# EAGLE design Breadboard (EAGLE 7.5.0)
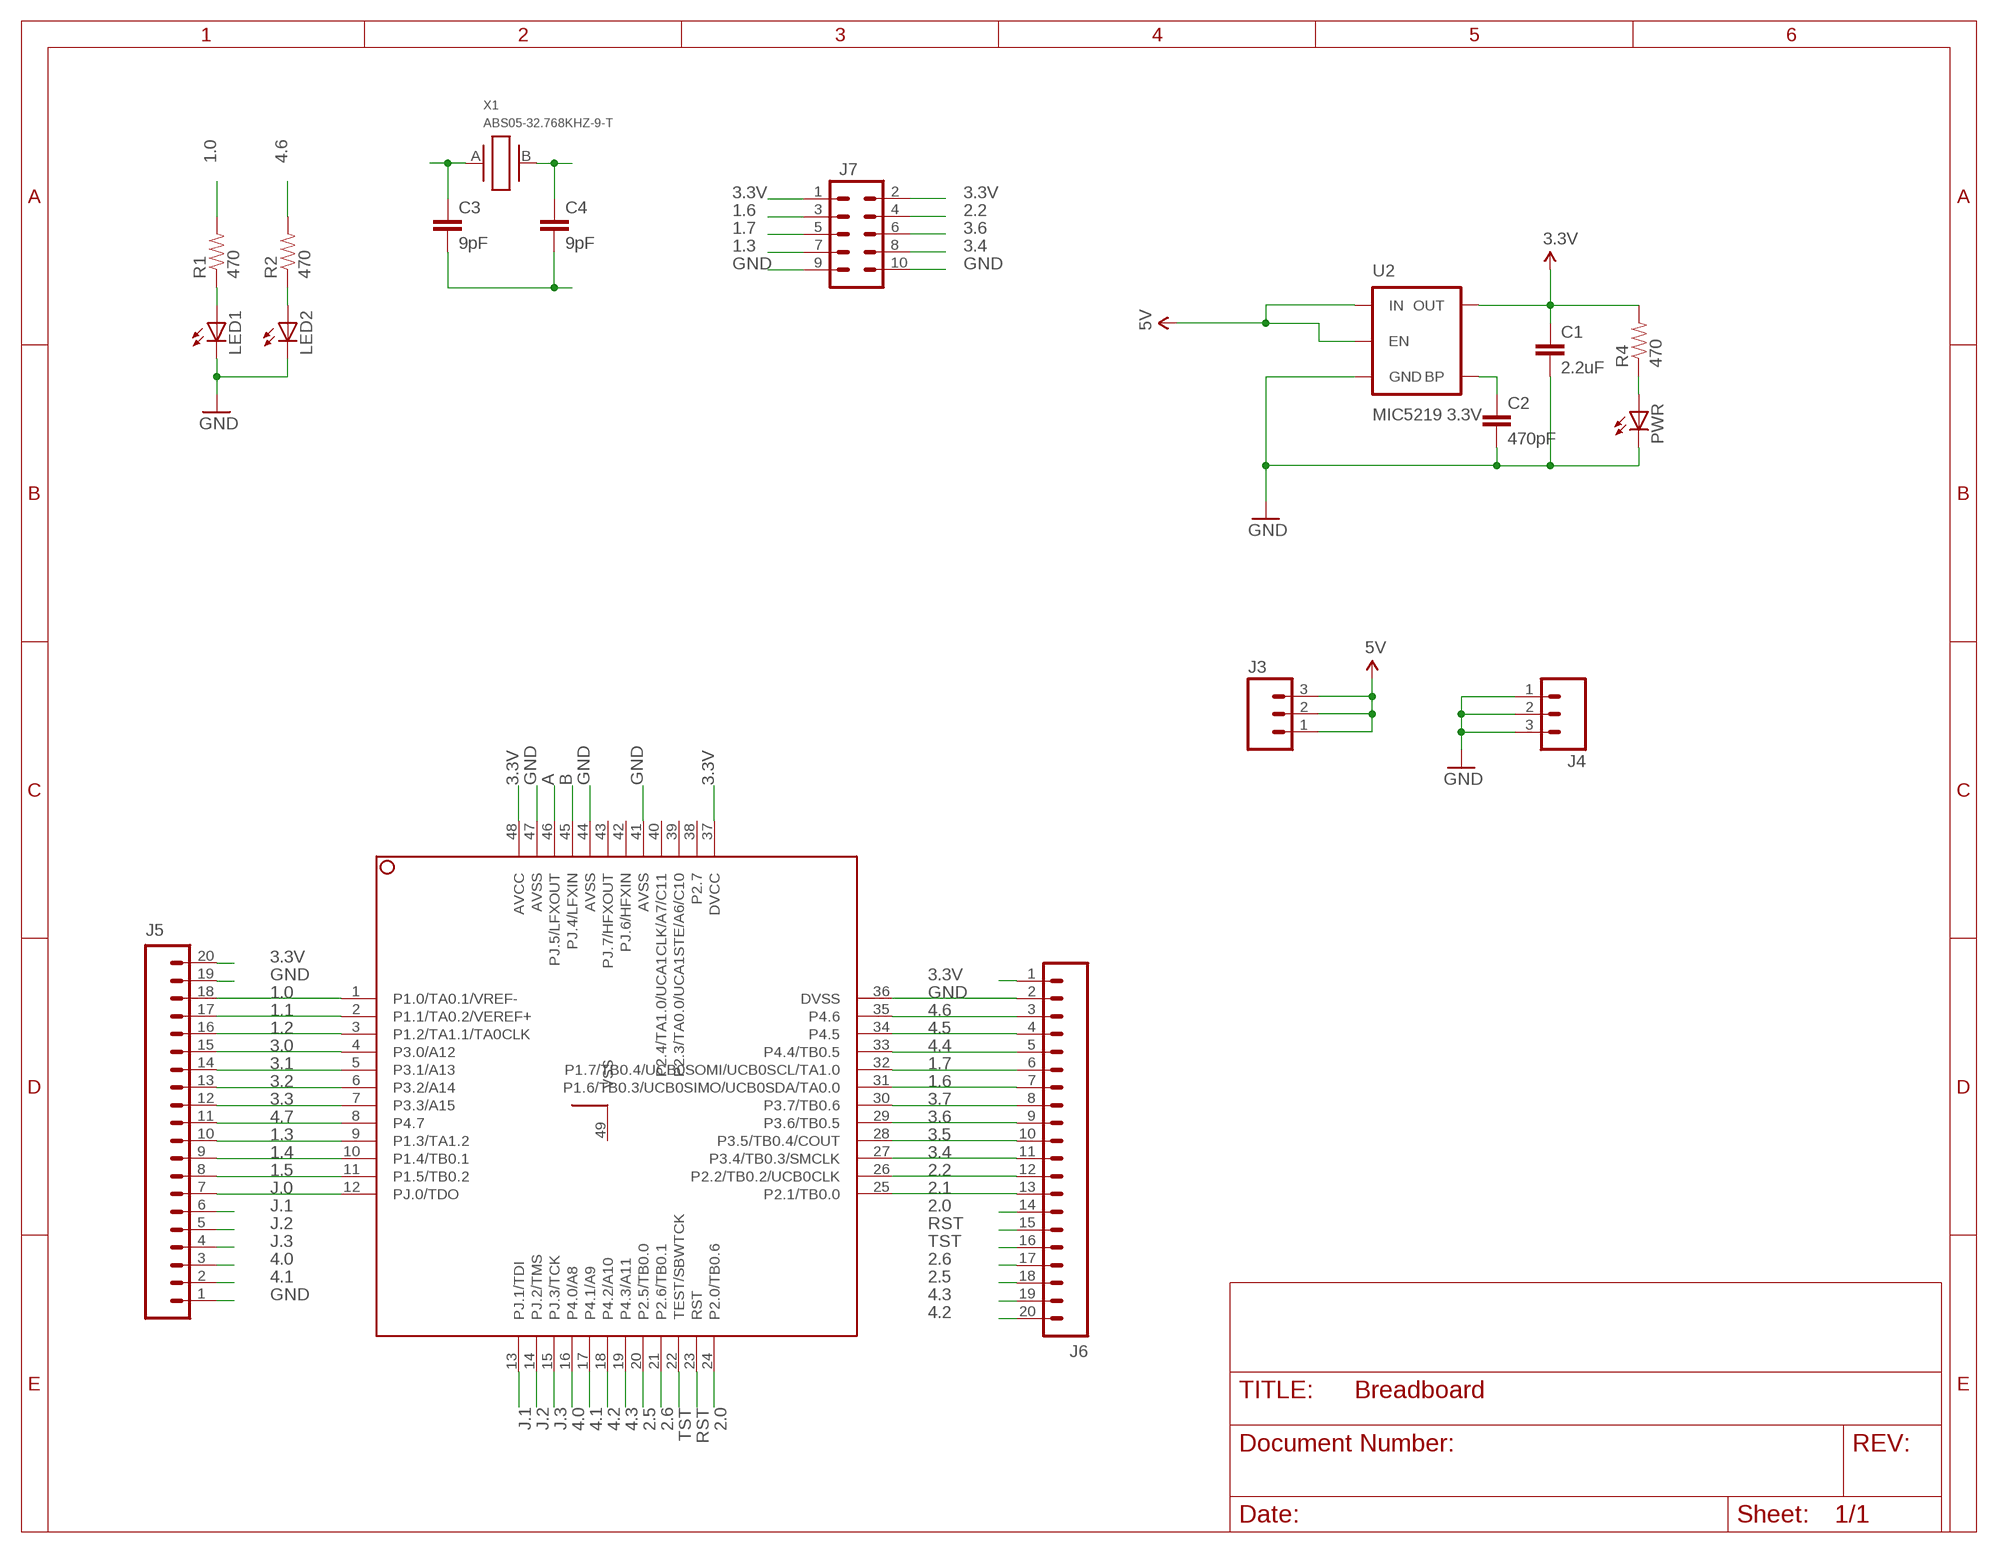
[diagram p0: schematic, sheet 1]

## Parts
C1  2.2uF  2.2UF-10V-20%(0603)  [0603-CAP]
C2  470pF  470PF-50V-5%(0603)SMD  [0603-CAP]
C3  9pF  9.0PF-50V-10%(0603)  [0603-CAP]
C4  9pF  9.0PF-50V-10%(0603)  [0603-CAP]
J3  M031X03_NO_SILK  [1X03_NO_SILK]
J4  M031X03_NO_SILK  [1X03_NO_SILK]
J5  M20NOSILK  [1X20_NOSILK]
J6  M20NOSILK  [1X20_NOSILK]
J7  M05X2NO_SILK  [2X5_NOSILK]
LED1  LEDCHIPLED_0805  [CHIPLED_0805]
LED2  LEDCHIPLED_0805  [CHIPLED_0805]
PWR  LEDCHIPLED_0805  [CHIPLED_0805]
R1  470  RESISTOR0805-RES  [0805]
R2  470  RESISTOR0805-RES  [0805]
R4  470  RESISTOR0805-RES  [0805]
U1  MSP430FR5969_RGZ_48  [RGZ48_4P1X4P1]
U2  MIC5219 3.3V  V_REG_MIC52193.3V  [SOT23-5]
X1  ABS05-32.768KHZ-9-T  [ABS05]

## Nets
1.0: J5.18 R1.2 U1.1(P1.0/TA0.1/VREF-)
1.1: J5.17 U1.2(P1.1/TA0.2/VEREF+)
1.2: J5.16 U1.3(P1.2/TA1.1/TA0CLK)
1.3: J5.10 J7.7 U1.9(P1.3/TA1.2)
1.4: J5.9 U1.10(P1.4/TB0.1)
1.5: J5.8 U1.11(P1.5/TB0.2)
1.6: J6.7 J7.3 U1.31(P1.6/TB0.3/UCB0SIMO/UCB0SDA/TA0.0)
1.7: J6.6 J7.5 U1.32(P1.7/TB0.4/UCB0SOMI/UCB0SCL/TA1.0)
2.0: J6.14 U1.24(P2.0/TB0.6)
2.1: J6.13 U1.25(P2.1/TB0.0)
2.2: J6.12 J7.4 U1.26(P2.2/TB0.2/UCB0CLK)
2.5: J6.18 U1.20(P2.5/TB0.0)
2.6: J6.17 U1.21(P2.6/TB0.1)
3.0: J5.15 U1.4(P3.0/A12)
3.1: J5.14 U1.5(P3.1/A13)
3.2: J5.13 U1.6(P3.2/A14)
3.3: J5.12 U1.7(P3.3/A15)
3.3V: C1.1 J5.20 J6.1 J7.1 J7.2 R4.2 U1.37(DVCC) U1.48(AVCC) U2.5(OUT)
3.4: J6.11 J7.8 U1.27(P3.4/TB0.3/SMCLK)
3.5: J6.10 U1.28(P3.5/TB0.4/COUT)
3.6: J6.9 J7.6 U1.29(P3.6/TB0.5)
3.7: J6.8 U1.30(P3.7/TB0.6)
4.0: J5.3 U1.16(P4.0/A8)
4.1: J5.2 U1.17(P4.1/A9)
4.2: J6.20 U1.18(P4.2/A10)
4.3: J6.19 U1.19(P4.3/A11)
4.4: J6.5 U1.33(P4.4/TB0.5)
4.5: J6.4 U1.34(P4.5)
4.6: J6.3 R2.2 U1.35(P4.6)
4.7: J5.11 U1.8(P4.7)
5V: J3.1 J3.2 J3.3 U2.1(IN) U2.3(EN)
A: C3.1 U1.46(PJ.5/LFXOUT) X1.A
B: C4.1 U1.45(PJ.4/LFXIN) X1.B
GND: C1.2 C2.2 C3.2 C4.2 J4.1 J4.2 J4.3 J5.1 J5.19 J6.2 J7.9 J7.10 LED1.C LED2.C PWR.C U1.36(DVSS) U1.41(AVSS) U1.44(AVSS) U1.47(AVSS) U2.2(GND)
J.0: J5.7 U1.12(PJ.0/TDO)
J.1: J5.6 U1.13(PJ.1/TDI)
J.2: J5.5 U1.14(PJ.2/TMS)
J.3: J5.4 U1.15(PJ.3/TCK)
N$1: LED2.A R2.1
N$2: PWR.A R4.1
N$4: LED1.A R1.1
N$7: C2.1 U2.4(BP)
RST: J6.15 U1.23(RST)
TST: J6.16 U1.22(TEST/SBWTCK)
Unconnected: U1.38(P2.7) U1.39(P2.3/TA0.0/UCA1STE/A6/C10) U1.40(P2.4/TA1.0/UCA1CLK/A7/C11) U1.42(PJ.6/HFXIN) U1.43(PJ.7/HFXOUT) U1.49(VSS)

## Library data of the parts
C1 = SparkFun-Capacitors:2.2UF-10V-20%(0603): CAP-07888; PROD_ID: CAP-07888
C2 = SparkFun-Capacitors:470PF-50V-5%(0603): CAP-07884; PROD_ID: CAP-07884
C3 C4 = SparkFun-Capacitors:9.0PF-50V-10%(0603): CAP-09341; PROD_ID: CAP-09341; VALUE: 9.0pF
J3 J4 = SparkFun-Connectors:M03: Header 3 Standard 3-pin 0.1" header. Use with straight break away headers (SKU : PRT-00116), right angle break away headers (PRT-00553), swiss pins (PRT-00743), machine pins (PRT-00117), and female headers (PRT-00115). Molex polarized connector foot print use with SKU : PRT-08232 with associated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
J5 J6 = SparkFun-Connectors:M20: 1x20 .1" header This is just like the LOCK variant in that the holes are staggared by 5 mil, but except for the last two holes. They are not altered from the "standard" footprint layout. This is used for a special purpose on the layout of our Graphic LCD Backpack. Make sure you want to use this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
J7 = SparkFun-Connectors:M05X2: Header 5x2 Standard 10-pin dual row 0.1" header. Commonly used with AVR-ISP. Use with Spark Fun Electronics SKU: PRT-00778
LED1 LED2 PWR = adafruit:LED: LED
R1 R2 R4 = SparkFun-Passives:RESISTOR: Resistor
U1 = msp430:MSP430FR5969_RGZ_48: MSP430FR59xx Mixed Signal Microcontroller Package: RGZ-S-PQVFN-N48 (MSP430FR596x and MSP430FR586x) Description The Texas Instruments MSP430FR58xx and MSP430FR59xx family of ultralow-power microcontrollers consists of several devices featuring embedded FRAM nonvolatile memory, an ultralow-power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; MANUFACTURER_PART_NUMBER: msp430fr5969_rgz_48; VENDOR: Texas Instruments
U2 = SparkFun-PowerIC:V_REG_MIC5219: V_REG MIC5219 Standard 3.3V and 5V 500mA LDO voltage regulator in SOT-23 layout. Micrel part MIC5219. BP (by-pass) pin is used to lower output noise with 470pF cap, may be left open.; PROD_ID: VREG-09872
X1 = abs05:ABS05-32.768KHZ: 32.768kHz Crystal; DIGIKEY: 535-11897-1-ND

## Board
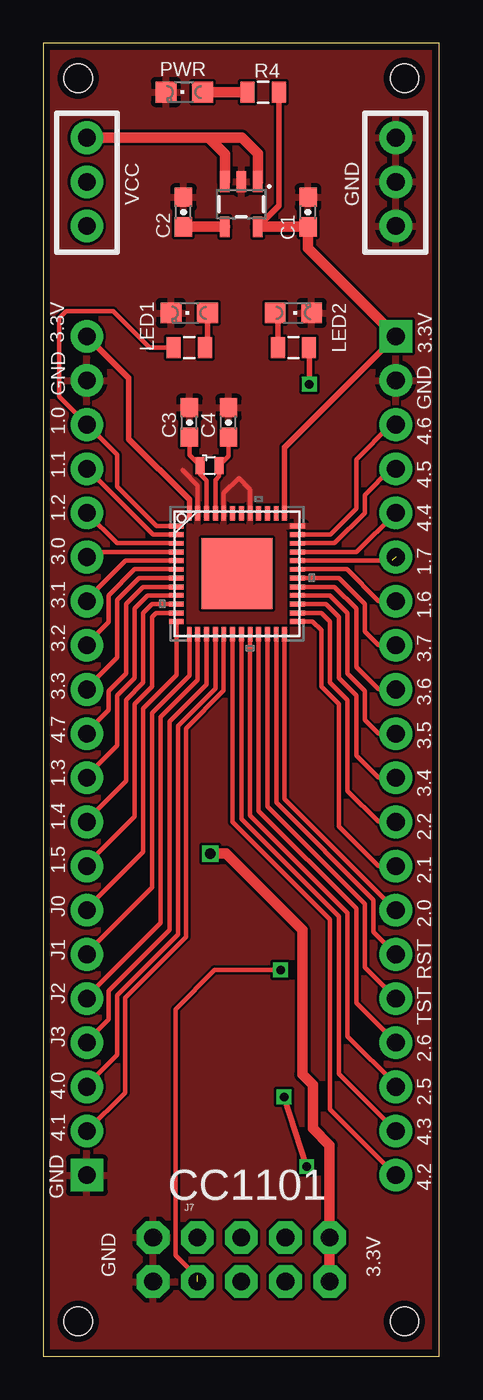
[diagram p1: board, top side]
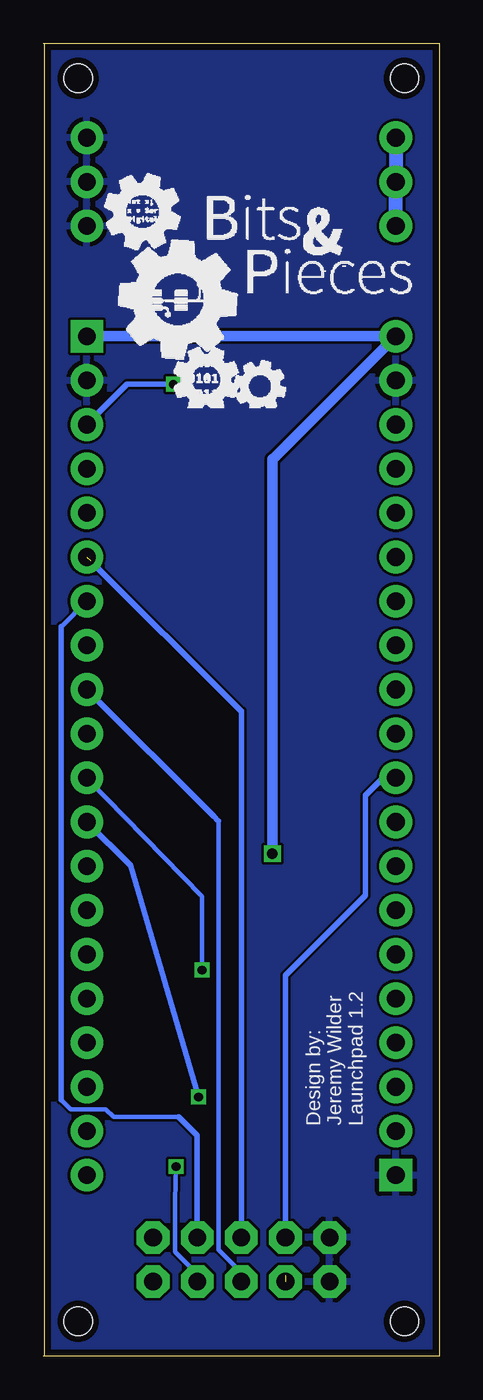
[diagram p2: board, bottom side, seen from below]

Size 22.78 x 75.5 mm. Coordinates in mm from the lower left corner, seen from the top.
Outline: 22.75,0 0,0 0,75.5 22.75,75.5
Outline: 22.75,0 22.78,0
Outline: 22.78,75.5 22.75,75.5
Outline: 22.75,75.5 22.75,0
Copper layers (1*16): Top 0.0356mm / dielectric 1.5011mm / Bottom 0.0356mm
Design rules "oshpark-2layer": minimum track width 6mil, minimum drill 13mil, track to track 6mil, track to pad 6mil, pad to pad 6mil, via to via 6mil, smd to smd 6mil, copper to edge 15mil, drill to drill 6mil, minimum pad ring 7mil, minimum via ring 7mil, stop-mask expansion 2.5mil, vias tented up to drill 0mil, thermal gap 10mil
Holes 1.6 mm at 2,73.5 20.78,73.5 2,2 20.78,2

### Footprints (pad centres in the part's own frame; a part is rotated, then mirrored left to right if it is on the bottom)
0603-CAP = smd 1.1 x 1: 1 -0.85,0; 2 0.85,0
1X03_NO_SILK = drill 1.016 pad 1.88: 1 0,0; 2 2.54,0; 3 5.08,0
1X20_NOSILK = drill 1.016 pad 1.88 square: 1 0,0 | drill 1.016 pad 1.88: 2 2.54,0; 3 5.08,0; 4 7.62,0; 5 10.16,0; 6 12.7,0; 7 15.24,0; 8 17.78,0; 9 20.32,0; 10 22.86,0; 11 25.4,0; 12 27.94,0; 13 30.48,0; 14 33.02,0; 15 35.56,0; 16 38.1,0; 17 40.64,0; 18 43.18,0; 19 45.72,0; 20 48.26,0
2X5_NOSILK = drill 1.016 pad 1.88 octagon: 1 -1.27,5.08; 2 1.27,5.08; 3 -1.27,2.54; 4 1.27,2.54; 5 -1.27,0; 6 1.27,0; 7 -1.27,-2.54; 8 1.27,-2.54; 9 -1.27,-5.08; 10 1.27,-5.08
CHIPLED_0805 = smd 1.2 x 1.2: A 0,-1.05; C 0,1.05
0805 = smd 0.8 x 1.2: 1 -0.9,0; 2 0.9,0
RGZ48_4P1X4P1 = smd 0.838 x 0.279: 1 -3.48,2.743; 2 -3.48,2.261; 3 -3.48,1.753; 4 -3.48,1.245; 5 -3.48,0.762; 6 -3.48,0.254; 7 -3.48,-0.254; 8 -3.48,-0.762; 9 -3.48,-1.245; 10 -3.48,-1.753; 11 -3.48,-2.261; 12 -3.48,-2.743; 25 3.48,-2.743; 26 3.48,-2.261; 27 3.48,-1.753; 28 3.48,-1.245; 29 3.48,-0.762; 30 3.48,-0.254; 31 3.48,0.254; 32 3.48,0.762; 33 3.48,1.245; 34 3.48,1.753; 35 3.48,2.261; 36 3.48,2.743 | smd 0.279 x 0.838: 13 -2.743,-3.48; 14 -2.261,-3.48; 15 -1.753,-3.48; 16 -1.245,-3.48; 17 -0.762,-3.48; 18 -0.254,-3.48; 19 0.254,-3.48; 20 0.762,-3.48; 21 1.245,-3.48; 22 1.753,-3.48; 23 2.261,-3.48; 24 2.743,-3.48; 37 2.743,3.48; 38 2.261,3.48; 39 1.753,3.48; 40 1.245,3.48; 41 0.762,3.48; 42 0.254,3.48; 43 -0.254,3.48; 44 -0.762,3.48; 45 -1.245,3.48; 46 -1.753,3.48; 47 -2.261,3.48; 48 -2.743,3.48 | smd 4.089 x 4.089: 49 0,0
SOT23-5 = smd 0.55 x 1.2: 1 -0.95,-1.3; 2 0,-1.3; 3 0.95,-1.3; 4 0.95,1.3; 5 -0.95,1.3
ABS05 = smd 0.5 x 1: A -0.55,0; B 0.55,0

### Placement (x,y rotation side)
C1  15.23,65.8 90 top
C2  8.05,65.8 90 top
C3  8.4,53.7 90 top
C4  10.65,53.7 90 top
J3  2.5,65 90 top
J4  20.28,70.08 270 top
J5  2.5,10.4 90 top
J6  20.28,58.66 270 top
J7  11.39,5.55 270 top
LED1  8.39,60 90 top
LED2  14.39,60 270 top
PWR  8.1,72.7 90 top
R1  8.39,58 180 top
R2  14.39,58 0 top
R4  12.65,72.7 0 top
U1  11.14,45 0 top
U2  11.39,66.25 180 top
X1  9.56,51.22 0 top

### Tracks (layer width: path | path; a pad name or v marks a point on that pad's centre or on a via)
1.0
  Top 0.254: U1.1 6.51,47.74 4.25,50 4.25,51.85 2.52,53.58 J5.18 2.5,53.6 0.9,55.2 0.9,59.7 1.3,60.1 4,60.1 6.1,58 R1.2
1.1
  Top 0.254: U1.2 6.3,47.26 2.52,51.04 J5.17
1.2
  Top 0.254: U1.3 4.25,46.75 J5.16
1.3
  Top 0.254: U1.9 6,43.76 5.25,43 5.25,39 4.25,38 4.25,35.11 2.5,33.36 J5.10
  Bottom 0.305: J7.7 8.85,21.9 4.25,26.5 4.25,32.25 3.22,33.28 2.52,33.28 J5.10
1.4
  Top 0.254: U1.10 6.25,43.25 5.75,42.75 5.75,38.75 4.75,37.75 4.75,33.07 2.5,30.82 J5.9
1.5
  Top 0.254: U1.11 6.49,42.74 6.25,42.5 6.25,38.5 5.25,37.5 5.25,31.03 2.5,28.28 J5.8
1.6
  Top 0.254: U1.31 17.46,45.25 19.27,43.44 20.26,43.44 J6.7
  Bottom 0.254: 15,13.75 18.75,13.75 19.2,14.2 21.2,14.2 21.75,14.75 | 21.75,41.97 21.73,41.97 J6.7
  Bottom 0.305: 21.75,14.75 21.75,41.97 | J7.3 13.93,12.68 15,13.75
1.7  (1 unrouted)
  Top 0.254: U1.32 20.06,45.76
  Bottom 0.305: J7.5 11.39,37.09 11.41,37.09 J6.6
2.0
  Top 0.254: U1.24 13.88,32.04 J6.14
2.1
  Top 0.254: U1.25 15.49,42.26 16,41.75 16,38.5 17,37.5 17,30.47 19.27,28.2 20.26,28.2 J6.13
2.2  (via drill 0.5)
  Top 0.254: U1.26 16.01,42.74 16.5,42.25 16.5,38.75 17.5,37.75 17.5,32.51 19.27,30.74 20.26,30.74 J6.12
  Top 0.305: v15.15,10.9 v13.85,14.9
  Bottom 0.254: J7.4 13.93,4.73 15.2,6 15.2,8.95 v15.15,10.9
  Bottom 0.305: v13.85,14.9 17.75,28.21 17.77,28.21 J6.12
2.5
  Top 0.254: U1.20 11.9,31.1 17.5,25.5 17.5,18.4 20.28,15.62 J6.18
2.6
  Top 0.254: U1.21 12.38,31.36 18,25.75 18,20.32 20.28,18.04 J6.17
3.0
  Top 0.254: U1.4 2.77,46.24 2.77,46.23 J5.15
3.1
  Top 0.254: U1.5 4.74,45.76 2.5,43.52 J5.14
3.2
  Top 0.254: U1.6 5.25,45.25 3.75,43.75 3.75,42.23 2.5,40.98 J5.13
3.3
  Top 0.254: U1.7 5.5,44.75 4.25,43.5 4.25,40.19 2.5,38.44 J5.12
3.3V  (via drill 0.6)
  Top 0.305: U1.37 13.88,52.28 13.9,52.28 J6.1 | U1.48 8.4,49.25 4.9,52.75 4.9,56.28 4.88,56.28 J5.20 | R4.2 13.55,66.16 U2.5
  Top 0.61: U2.5 C1.1 | C1.1 | C1.1 15.23,63.73 20.28,58.68 J6.1 | J7.2 J7.1 16.47,12.13 15.5,13.1 15.5,15.6 14.9,16.2 14.9,24.5 10.5,28.9 v9.6,28.9
  Bottom 0.61: v9.6,28.9 9.6,51.58 9.58,51.58 J5.20 J6.1
3.4  (via drill 0.5)  (1 unrouted)
  Top 0.254: U1.27 16.25,43.25 17,42.5 17,39 18,38 18,34.55 19.27,33.28 20.26,33.28 J6.11 | 8.85,4.65 8.75,4.65 7.6,5.8 7.6,19.95 9.85,22.2 v13.65,22.2
  Bottom 0.254: v13.65,22.2 13.65,26.43 J6.11
3.5
  Top 0.254: U1.28 16.5,43.76 17.5,42.75 17.5,39.25 18.5,38.25 18.5,36.59 19.27,35.82 20.26,35.82 J6.10
3.6
  Top 0.254: U1.29 16.76,44.24 18,43 18,39.63 19.27,38.36 20.26,38.36 J6.9
  Bottom 0.254: J7.6 11.39,4.99 11.59,4.99 12.7,6.1 12.7,30.76 12.97,31.03
  Bottom 0.305: 12.7,30.78 12.72,30.78 12.97,31.03 J6.9
3.7
  Top 0.254: U1.30 17,44.75 18.5,43.25 18.5,41.67 19.27,40.9 20.26,40.9 J6.8
4.0
  Top 0.254: U1.16 9.89,38.4 7.75,36.25 7.75,24.25 4.25,20.75 4.25,17.33 2.5,15.58 J5.3
4.1
  Top 0.254: U1.17 10.38,38.28 8.2,36.1 8.2,24.1 4.7,20.6 4.7,15.14 J5.2
4.2
  Top 0.254: U1.18 10.89,30.71 16.5,25.1 16.5,14.18 J6.20
4.3
  Top 0.254: U1.19 11.39,30.91 17,25.3 17,16.22 J6.19
4.4
  Top 0.254: U1.33 18.02,46.24 J6.5
4.5
  Top 0.254: U1.34 16.75,46.75 18.5,48.5 18.5,49.53 20.01,51.04 J6.4
4.6  (via drill 0.5)
  Top 0.254: U1.35 16.51,47.26 18,48.75 18,51.57 20.01,53.58 J6.3
  Top 0.305: v15.3,55.9 R2.2
  Bottom 0.305: v15.3,55.9 17.96,55.9 J6.3
4.7
  Top 0.254: U1.8 5.74,44.24 4.75,43.25 4.75,39.25 3.75,38.25 3.75,37.15 2.5,35.9 J5.11
5V
  Top 0.61: U2.1 12.34,69.16 11.42,70.08 9.5,70.08 | 9.5,70.08 J3.3 | U2.3 10.44,69.14 9.5,70.08
  Bottom 0.813: J3.1 J3.2 J3.3
A
  Top 0.254: U1.46 9.39,50.36 9.01,50.74 X1.A 8.4,51.83 C3.1
B
  Top 0.254: U1.45 9.89,50.4 10.11,50.61 X1.B 10.65,51.76 C4.1
GND
  Top 0.254: U1.41 11.9,49.85 11.25,50.5 10.38,49.63 U1.44 | U1.47 8.88,50.07 8,50.95
  pour Bottom: 0,75.5 22.78,75.5 22.78,0 0,0
  pour Top: 0.02,75.5 22.78,75.5 22.78,0 0.27,0
J.0
  Top 0.254: U1.12 7.66,39.16 5.75,37.25 5.75,28.99 2.5,25.74 J5.7
J.1
  Top 0.254: U1.13 8.4,39.15 6.25,37 6.25,26.95 2.5,23.2 J5.6
J.2
  Top 0.254: U1.14 8.88,38.88 6.75,36.75 6.75,24.91 2.5,20.66 J5.5
J.3
  Top 0.254: U1.15 9.39,38.64 7.25,36.5 7.25,24.5 3.75,21 3.75,19.37 2.5,18.12 J5.4
N$1
  Top 0.305: R2.1 13.49,59.85 LED2.A
N$2
  Top 0.61: R4.1 PWR.A
N$4
  Top 0.305: LED1.A 9.44,58.15 R1.1
N$7
  Top 0.61: 7.95,64.95 C2.1 U2.4
RST
  Top 0.254: U1.23 13.4,31.85 19,26.25 19,24.4 20.28,23.12 J6.15
TST
  Top 0.254: U1.22 12.89,31.61 18.5,26 18.5,22.36 20.28,20.58 J6.16

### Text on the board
tPlace: GND | BREAKOUT / POWER | VCC | 3.3V | 3.3V | GND | GND | 4.6 | 1.0 | 4.5 | 1.1 | 4.4 | 1.2 | 3.0 | 1.7 | 1.6 | 3.1 | 3.7 | 3.2 | 3.6 | 3.3 | 3.5 | 4.7 | 3.4 | 1.3 | 2.2 | 1.4 | 2.1 | 1.5 | 2.0 | J0 | RST | J1 | TST | J2 | J3 | 2.6 | 2.5 | 4.0 | 4.3 | 4.1 | CC1101 | 4.2 | GND | GND | 3.3V
bPlace: Design by: / Jeremy Wilder / Launchpad 1.2

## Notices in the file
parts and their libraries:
SparkFun-Connectors: Licensing: Creative Commons ShareAlike 4.0 International - https://creativecommons.org/licenses/by-sa/4.0
